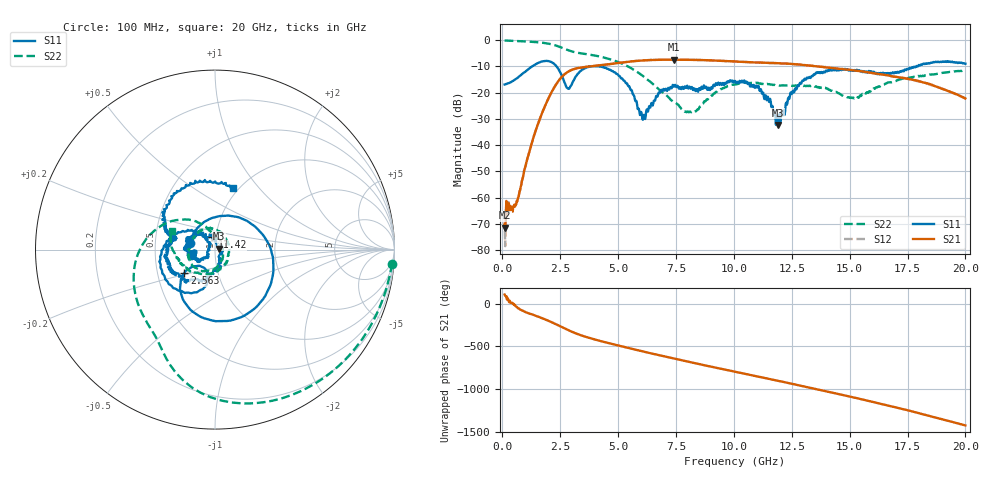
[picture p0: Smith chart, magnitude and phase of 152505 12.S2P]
!  2-Port S-parameters saved by WinCal
! VAR MeasName=S-Parameters (CALIBRATED_DATA) read from VNA (N5230C)
! VAR MeasDate=4/10/2015 9:29:29 AM
! VAR NAME=152505 12
! VAR FILENAME=152505 12.S2P
! VAR DATE=4/10/2015 9:29:30 AM
! VAR PHYS_PORTS=1,2
# Hz S DB R 50
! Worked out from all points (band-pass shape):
!   801 points, 100 MHz to 20 GHz, reference 50 ohm
!   highest |S21| = -7.40 dB at 7.413 GHz (marker M1); lowest = -71.5 dB at 124.9 MHz (marker M2)
!   |S21| within 3 dB of the highest: 3.424 GHz to 14.05 GHz (10.62 GHz wide, 122 % of centre)
!   lowest |S11| = -32.3 dB at 11.92 GHz (marker M3), VSWR 1.05, Z = 52.4 + j0.627 ohm
!   |S11| at or under -10 dB: start of sweep to 1.283 GHz; 2.345 GHz to 3.754 GHz (1.41 GHz wide, 46.2 % of centre); 4.266 GHz to 17.87 GHz (13.6 GHz wide, 123 % of centre)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
!   |S22| runs from -27.5 to -0.1 dB; largest |S21 - S12| = 0.007
!   S11 on the Smith chart (normalised r, x): 100 MHz: 0.76, +0.06; 2.563 GHz: 0.69, -0.19; 11.42 GHz: 0.96, +0.13; 20 GHz: 0.94, +0.74
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1e8  -16.88 164.3  -70.24 106.7  -67.85 69.6  -0.08 -4.6
1.24875e8  -16.83 160.2  -71.48 89.8  -78.51 67.1  -0.11 -5.5
6.4725e8  -14.39 79.4  -61.43 -45.9  -61.30 -46.2  -0.31 -26.3
1.3935e9  -9.41 -16.3  -35.74 -137.2  -35.78 -137.1  -0.67 -56.6
1.965625e9  -7.94 -83.5  -22.66 162.2  -22.69 162.4  -1.26 -81.4
2.562625e9  -13.36 -142.8  -14.05 86.4  -14.06 86.4  -2.82 -107.3
2.861125e9  -18.54 -120.9  -11.91 47.8  -11.89 48.0  -3.85 -116.7
3.43325e9  -11.35 -117.3  -10.40 -14.0  -10.37 -13.7  -5.04 -131.7
4.950625e9  -12.86 154.9  -8.73 -126.8  -8.71 -127.1  -8.11 172.9
6.07e9  -30.35 153.9  -7.71 160.0  -7.68 160.0  -13.60 128.3
6.741625e9  -20.18 -146.4  -7.45 117.2  -7.43 116.9  -18.53 108.2
7.41325e9  -17.68 -158.8  -7.40 76.1  -7.39 76.0  -23.54 84.3
8.06e9  -18.15 -173.0  -7.46 37.5  -7.44 37.4  -27.48 27.0
8.681875e9  -17.88 -173.5  -7.57 0.7  -7.55 0.5  -24.05 -47.0
1.005e10  -15.49 174.6  -8.09 -78.4  -8.12 -78.7  -16.83 -130.1
1.141812e10  -22.87 104.2  -8.63 -155.9  -8.63 -155.8  -16.65 -179.0
1.191562e10  -32.26 14.2  -8.77 175.2  -8.79 175.4  -17.21 171.1
1.338325e10  -13.59 -124.0  -9.76 87.9  -9.67 88.0  -17.51 131.1
1.480112e10  -10.90 -172.1  -11.12 3.2  -11.05 2.1  -21.58 39.0
1.669162e10  -12.84 165.7  -13.47 -116.3  -13.54 -117.3  -16.11 -115.5
1.83085e10  -8.82 141.5  -16.41 133.2  -16.29 131.9  -13.46 -167.2
2e10  -8.95 74.1  -22.19 11.7  -22.24 12.5  -11.59 156.8
